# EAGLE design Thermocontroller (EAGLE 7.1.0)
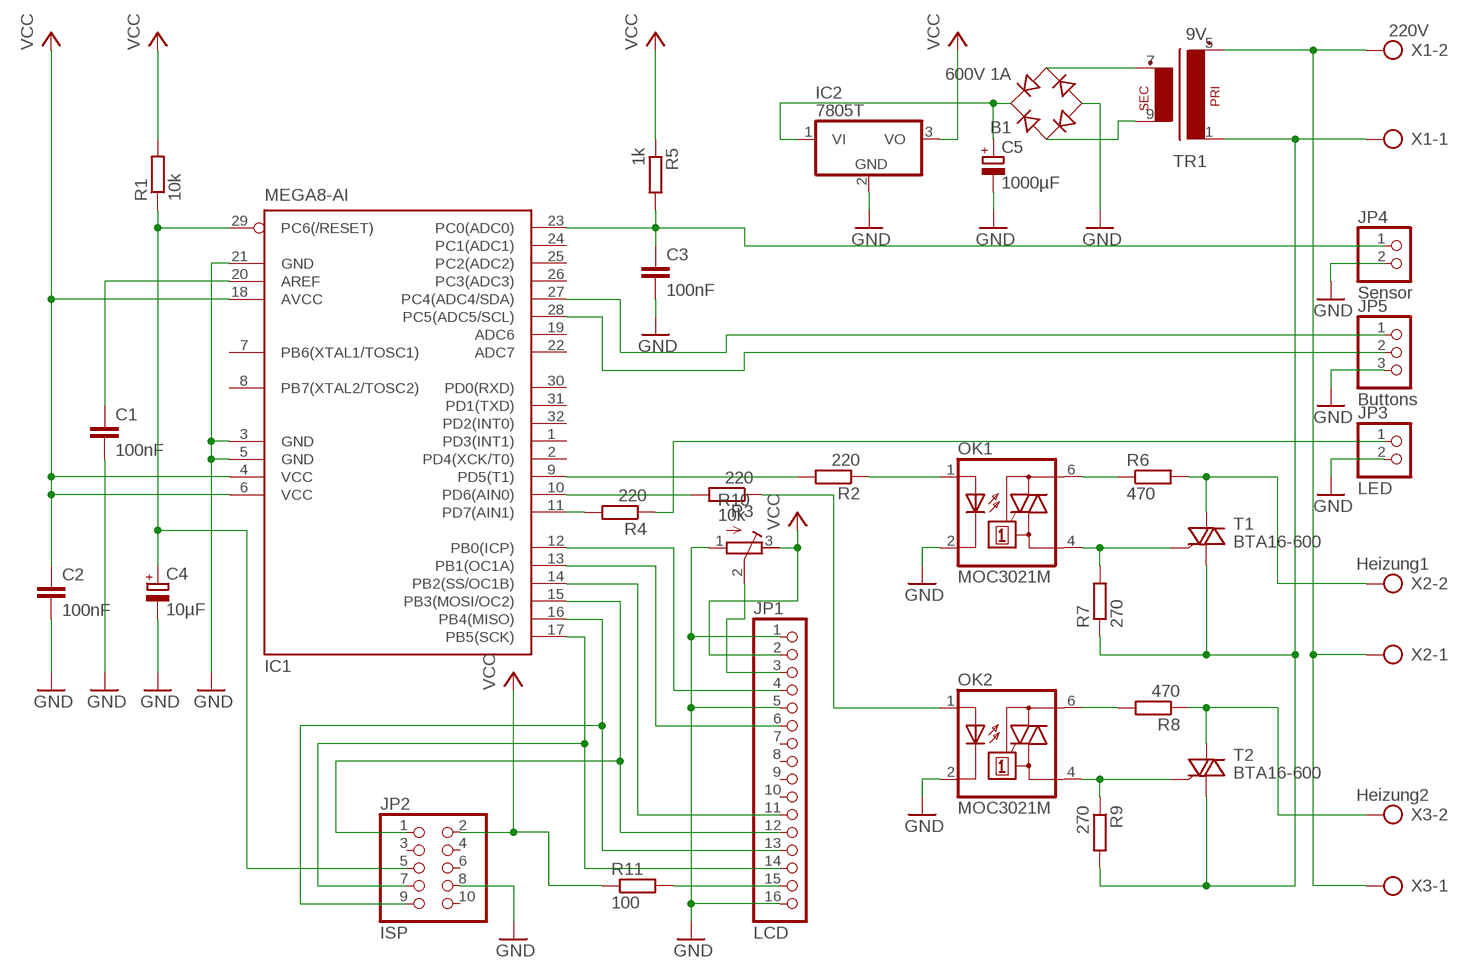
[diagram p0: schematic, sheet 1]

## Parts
B1  600V 1A  RB1A  [RB1A]
C1  100nF  C-EUC1206  [C1206]
C2  100nF  C-EUC0805  [C0805]
C3  100nF  C-EUC0805  [C0805]
C4  10µF  CPOL-EUSMCB  [SMC_B]
C5  1000µF  CPOL-EUE7.5-16  [E7,5-16]
IC1  MEGA8-AI  [TQFP32-08]
IC2  7805T  [TO220H]
JP1  LCD  PINHD-1X16  [1X16]
JP2  ISP  PINHD-2X5  [2X05]
JP3  LED  PINHD-1X2  [1X02]
JP4  Sensor  PINHD-1X2  [1X02]
JP5  Buttons  PINHD-1X3  [1X03]
OK1  MOC3021M  [DIL06]
OK2  MOC3021M  [DIL06]
R1  10k  R-EU_R1206  [R1206]
R2  220  R-EU_R1206  [R1206]
R3  220  R-EU_R1206  [R1206]
R4  220  R-EU_R1206  [R1206]
R5  1k  R-EU_R1206  [R1206]
R6  470  R-EU_0207/10  [0207/10]
R7  270  R-EU_0207/10  [0207/10]
R8  470  R-EU_0207/10  [0207/10]
R9  270  R-EU_0207/10  [0207/10]
R10  10k  R-TRIMM64Y  [RTRIM64Y]
R11  100  R-EU_0207/10  [0207/10]
T1  BTA16-600  BT138-V  [TO220BV]
T2  BTA16-600  BT138-V  [TO220BV]
TR1  9V  EI30-1  [EI30-1]
X1  220V  AK500/2  [AK500/2]
X2  Heizung1  AK500/2  [AK500/2]
X3  Heizung2  AK500/2  [AK500/2]

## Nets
GND: B1.- C1.2 C2.2 C3.2 C4.- C5.- IC1.3(GND) IC1.5(GND) IC1.21(GND) IC2.2(GND) JP1.1 JP1.5 JP1.16 JP2.8 JP3.2 JP4.2 JP5.3 OK1.2(C) OK2.2(C) R10.1(A)
N$1: TR1.5(P2) X1.2 X2.1 X3.1
N$2: B1.AC2 TR1.7(S3)
N$4: B1.AC1 TR1.9(S4)
N$5: B1.+ C5.+ IC2.1(VI)
N$6: OK2.6(A2) R8.2
N$7: OK1.6(A2) R6.1
N$8: OK2.4(A1) R9.1 T2.G
N$9: OK1.4(A1) R7.2 T1.G
N$13: R8.1 T2.T2(A2) X3.2
N$14: OK1.1(A) R2.1
N$15: IC1.9(PD5(T1)) R2.2
N$16: IC1.10(PD6(AIN0)) R3.2
N$17: OK2.1(A) R3.1
N$18: JP3.1 R4.1
N$19: IC1.11(PD7(AIN1)) R4.2
N$20: IC1.17(PB5(SCK)) JP1.14 JP2.7
N$21: IC1.16(PB4(MISO)) JP1.13 JP2.9
N$22: IC1.15(PB3(MOSI/OC2)) JP1.12 JP2.1
N$23: IC1.14(PB2(SS/OC1B)) JP1.11
N$24: IC1.13(PB1(OC1A)) JP1.6
N$25: IC1.12(PB0(ICP)) JP1.4
N$26: C3.1 IC1.23(PC0(ADC0)) JP4.1 R5.2
N$27: IC1.27(PC4(ADC4/SDA)) JP5.1
N$28: IC1.28(PC5(ADC5/SCL)) JP5.2
N$29: R7.1 R9.2 T1.T1(A1) T2.T1(A1) TR1.1 X1.1
N$30: C1.1 IC1.20(AREF)
N$31: C4.+ IC1.29(PC6(/RESET)) JP2.5 R1.1
N$32: R6.2 T1.T2(A2) X2.2
N$35: JP1.3 R10.2(S)
N$38: JP1.15 R11.2
VCC: C2.1 IC1.4(VCC) IC1.6(VCC) IC1.18(AVCC) IC2.3(VO) JP1.2 JP2.2 R1.2 R5.1 R10.3(E) R11.1
Unconnected: IC1.1(PD3(INT1)) IC1.2(PD4(XCK/T0)) IC1.7(PB6(XTAL1/TOSC1)) IC1.8(PB7(XTAL2/TOSC2)) IC1.19(ADC6) IC1.22(ADC7) IC1.24(PC1(ADC1)) IC1.25(PC2(ADC2)) IC1.26(PC3(ADC3)) IC1.30(PD0(RXD)) IC1.31(PD1(TXD)) IC1.32(PD2(INT0)) JP1.7 JP1.8 JP1.9 JP1.10 JP2.3 JP2.4 JP2.6 JP2.10

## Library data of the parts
B1 = rectifier:RB1A: RECTIFIER 1 A
C1-C3 = rcl:C-EU: CAPACITOR, European symbol
C4 C5 = rcl:CPOL-EU: POLARIZED CAPACITOR, European symbol
IC1 = atmel:MEGA8: MICROCONTROLLER 8 Kbytes FLASH, 1 kbytes SRAM, 512 bytes EEPROM, USART, 6-channel 10 bit ADC, 2-channel 8 bit ADC Pin compatible with Atmega48, ATMega88, ATMega168 Source: avr.lbr; MPN: ATMEGA8-16AU; OC_FARNELL: 9171371; OC_NEWARK: 73M8863
IC2 = linear:78*: Positive VOLTAGE REGULATOR Source: http://cache.national.com/ds/LM/LM78L05.pdf http://www.fairchildsemi.com/ds/LM/LM7805.pdf
JP1 = pinhead:PINHD-1X16: PIN HEADER
JP2 = pinhead:PINHD-2X5: PIN HEADER
JP3 JP4 = pinhead:PINHD-1X2: PIN HEADER
JP5 = pinhead:PINHD-1X3: PIN HEADER
OK1 OK2 = optocoupler:MOC30*M: RANDOM-PHASE OPTOISOLATORS TRIAC DRIVER OUTPUT Source: http://www.fairchildsemi.com MOC3020-M.pdf; MF: FAIRCHILD SEMICONDUCTOR; MPN: MOC3021-M; OC_FARNELL: 1021365; OC_NEWARK: 95B7895
R1-R9 R11 = rcl:R-EU_: RESISTOR, European symbol
R10 = rcl:R-TRIMM: Trimm resistor
T1 T2 = triac:BT138: TRIAC Source: http://www.semiconductors.philips.com BT138_SERIES_2.pdf
TR1 = trafo:EI30-1: TRANSFORMER 1 primary winding, 1 secondary winding ERA
X1-X3 = con-ptr500:AK500/2: CONNECTOR; OC_FARNELL: unknown; OC_NEWARK: unknown

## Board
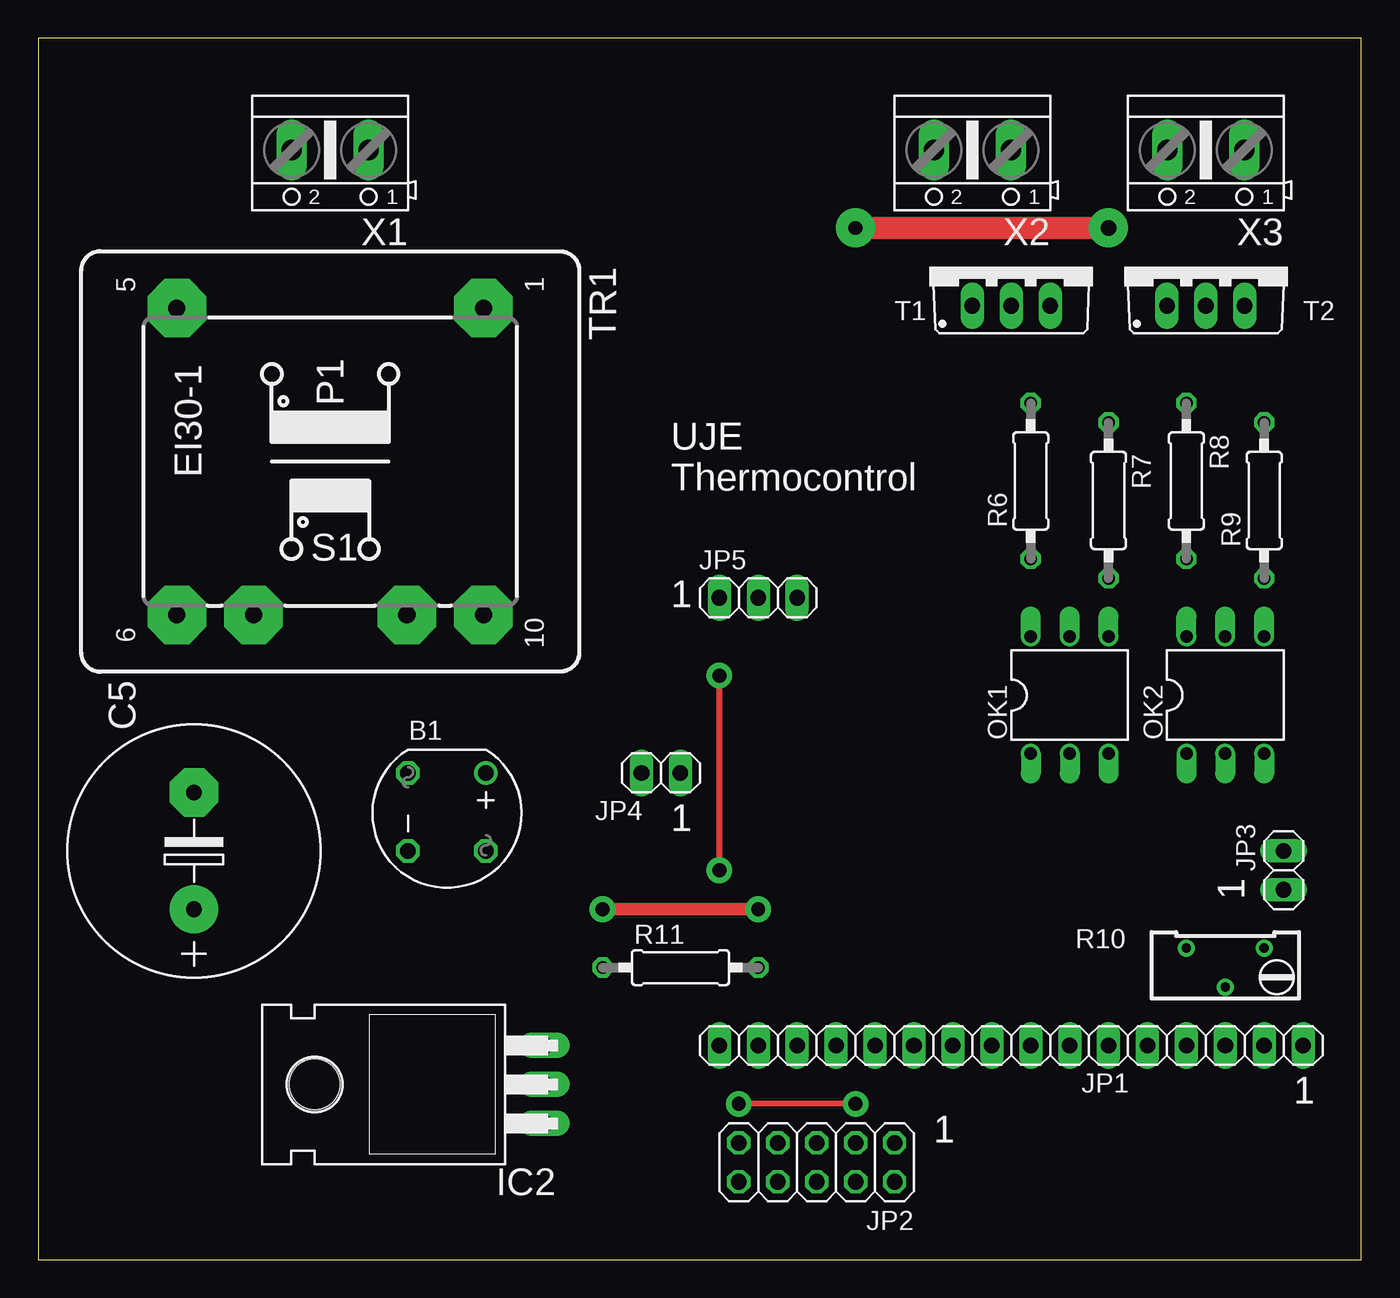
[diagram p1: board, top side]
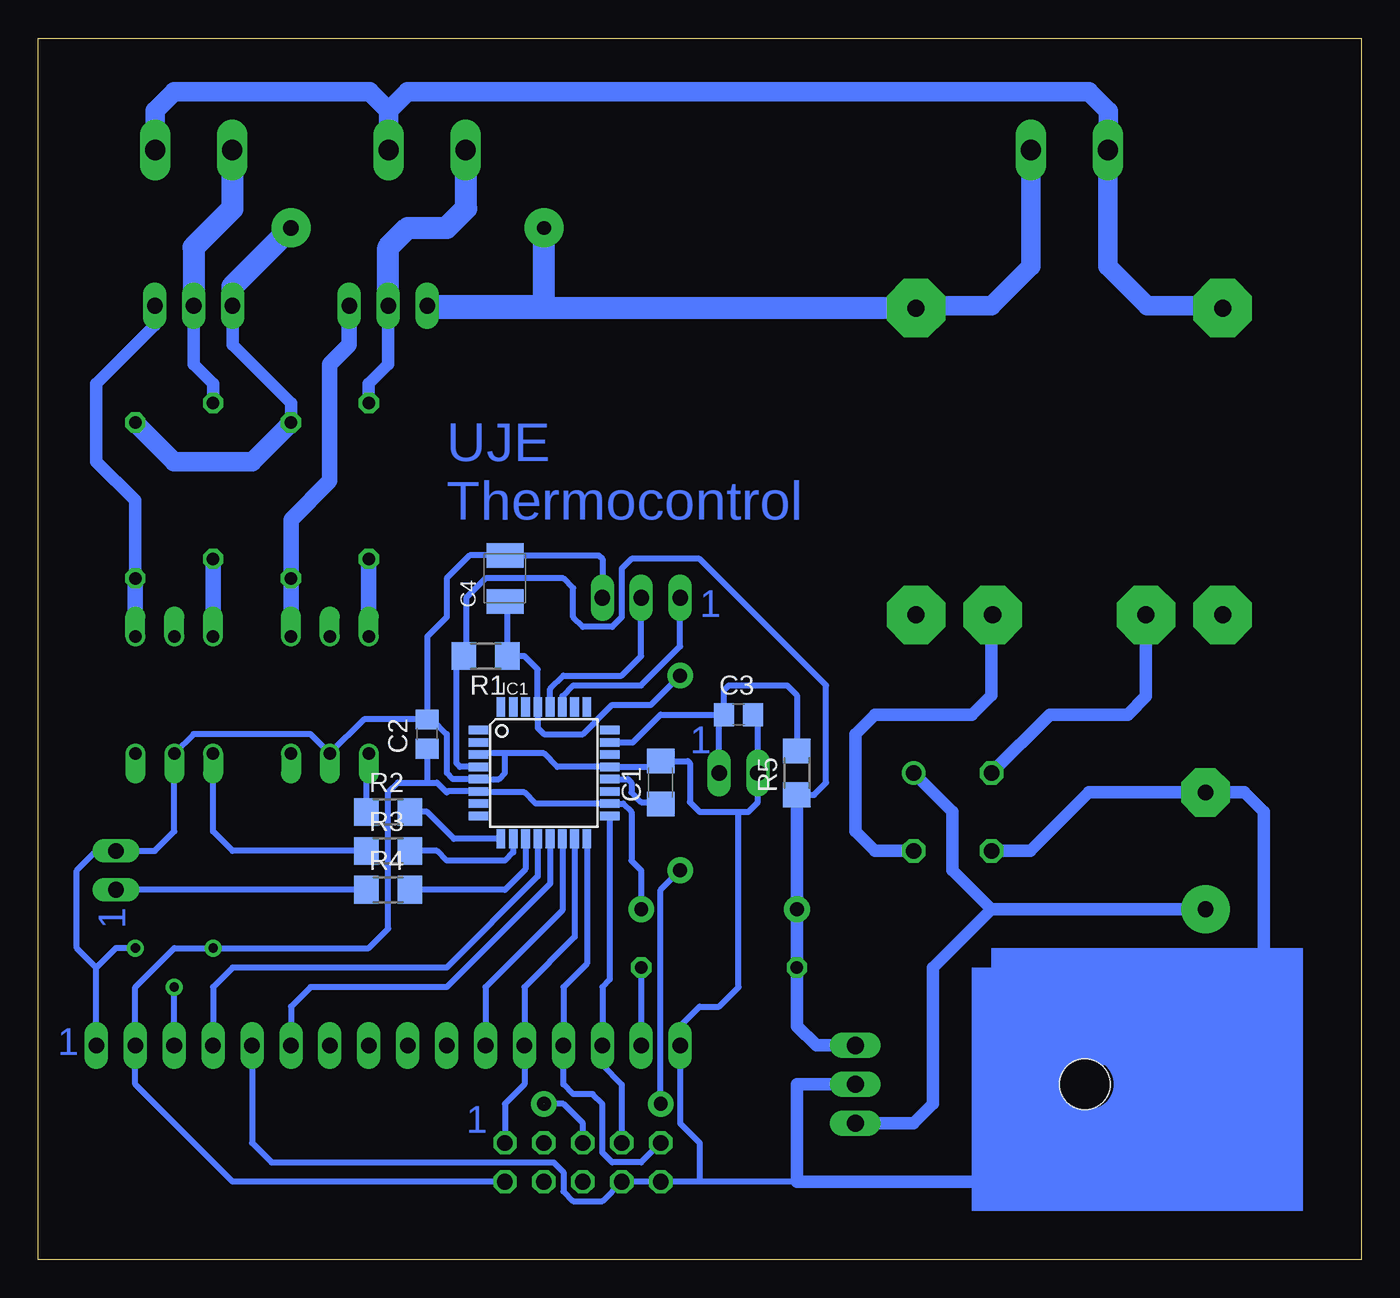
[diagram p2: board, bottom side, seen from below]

Size 86.34 x 79.68 mm. Coordinates in mm from the lower left corner, seen from the top.
Outline: 0,0 86.34,0 86.34,79.68 0,79.68 0,0
Copper layers (1*16): Top 0.035mm / dielectric 1.5mm / Bottom 0.035mm
Design rules "default": minimum track width 10mil, minimum drill 24mil, track to track 8mil, track to pad 8mil, pad to pad 8mil, via to via 8mil, smd to smd 8mil, copper to edge 40mil, drill to drill 8mil, minimum pad ring 10mil, minimum via ring 8mil, stop-mask expansion 4mil, vias tented up to drill 0mil, thermal gap 10mil

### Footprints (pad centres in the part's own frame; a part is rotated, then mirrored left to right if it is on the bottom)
RB1A = drill 1.016: + -2.54,2.54 | drill 1.016 octagon: - 2.54,-2.54; AC1 2.54,2.54; AC2 -2.54,-2.54
C1206 = smd 1.6 x 1.8: 1 -1.4,0; 2 1.4,0
C0805 = smd 1.3 x 1.5: 1 -0.95,0; 2 0.95,0
SMC_B = smd 1.6 x 2.4: + -1.5,0; - 1.5,0
E7,5-16 = drill 1.016 pad 3.15: + -3.81,0 | drill 1.016 pad 3.15 octagon: - 3.81,0
TQFP32-08 = smd 1.27 x 0.559: 1 -4.293,2.8; 2 -4.293,2; 3 -4.293,1.2; 4 -4.293,0.4; 5 -4.293,-0.4; 6 -4.293,-1.2; 7 -4.293,-2; 8 -4.293,-2.8; 17 4.293,-2.8; 18 4.293,-2; 19 4.293,-1.2; 20 4.293,-0.4; 21 4.293,0.4; 22 4.293,1.2; 23 4.293,2; 24 4.293,2.8 | smd 0.559 x 1.27: 9 -2.8,-4.293; 10 -2,-4.293; 11 -1.2,-4.293; 12 -0.4,-4.293; 13 0.4,-4.293; 14 1.2,-4.293; 15 2,-4.293; 16 2.8,-4.293; 25 2.8,4.293; 26 2,4.293; 27 1.2,4.293; 28 0.4,4.293; 29 -0.4,4.293; 30 -1.2,4.293; 31 -2,4.293; 32 -2.8,4.293
TO220H = drill 1.118 long: 1 -2.54,-10.16; 2 0,-10.16; 3 2.54,-10.16 | hole 3.302: 0,4.826
1X16 = drill 1.016 long: 1 -19.05,0; 2 -16.51,0; 3 -13.97,0; 4 -11.43,0; 5 -8.89,0; 6 -6.35,0; 7 -3.81,0; 8 -1.27,0; 9 1.27,0; 10 3.81,0; 11 6.35,0; 12 8.89,0; 13 11.43,0; 14 13.97,0; 15 16.51,0; 16 19.05,0
2X05 = drill 1.016 octagon: 1 -5.08,-1.27; 2 -5.08,1.27; 3 -2.54,-1.27; 4 -2.54,1.27; 5 0,-1.27; 6 0,1.27; 7 2.54,-1.27; 8 2.54,1.27; 9 5.08,-1.27; 10 5.08,1.27
1X02 = drill 1.016 long: 1 -1.27,0; 2 1.27,0
1X03 = drill 1.016 long: 1 -2.54,0; 2 0,0; 3 2.54,0
DIL06 = drill 0.813 offset: 1 -2.54,-3.81; 2 0,-3.81; 3 2.54,-3.81; 4 2.54,3.81; 5 0,3.81; 6 -2.54,3.81
R1206 = smd 1.6 x 1.803: 1 -1.422,0; 2 1.422,0
0207/10 = drill 0.813 octagon: 1 -5.08,0; 2 5.08,0
RTRIM64Y = drill 0.61: 1 0,-2.54; 2 -2.54,0; 3 0,2.54
TO220BV = drill 1.016 long: G 2.54,-2.54; T1 -2.54,-2.54; T2 0,-2.54
EI30-1 = drill 1.118 pad 3.81 octagon: 1 -10.008,10.008; 5 -10.008,-10.008; 6 10.008,-10.008; 7 10.008,-5.004; 9 10.008,5.004; 10 10.008,10.008
AK500/2 = drill 1.321 long: 1 -2.515,0; 2 2.515,0

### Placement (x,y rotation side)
B1  26.67,29.21 270 top
C1  45.72,31.12 90 bottom
C2  60.96,34.29 90 bottom
C3  40.64,35.56 0 bottom
C4  55.88,44.45 90 bottom
C5  10.16,26.67 90 top
IC1  53.34,31.75 0 bottom
IC2  22.86,11.43 90 top
JP1  63.5,13.97 180 top
JP2  50.8,6.35 180 top
JP3  81.28,25.4 90 top
JP4  40.64,31.75 180 top
JP5  46.99,43.18 0 top
OK1  67.31,36.83 0 top
OK2  77.47,36.83 0 top
R1  57.15,39.37 180 bottom
R2  63.5,29.21 0 bottom
R3  63.5,26.67 0 bottom
R4  63.5,24.13 0 bottom
R5  36.83,31.75 90 bottom
R6  64.77,50.8 90 top
R7  69.85,49.53 270 top
R8  74.93,50.8 270 top
R9  80.01,49.53 90 top
R10  77.47,20.32 90 top
R11  41.91,19.05 0 top
T1  63.5,64.77 0 top
T2  76.2,64.77 0 top
TR1  19.05,52.07 270 top
X1  19.05,72.39 180 top
X2  60.96,72.39 180 top
X3  76.2,72.39 180 top

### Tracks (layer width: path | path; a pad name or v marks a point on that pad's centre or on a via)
GND
  Bottom 0.406: JP1.1 82.55,19.05 | 82.55,19.05 83.82,20.32 83.82,25.4 82.55,26.67 JP3.2 78.74,26.67 77.47,27.94 OK2.2 76.2,34.29 68.58,34.29 OK1.2 65.09,35.24 C2.2 | R10.1 81.28,20.32 82.55,19.05 | 55.88,33.02 53.34,33.02 52.47,32.15 IC1.21 46.09,32.15 C1.2 43.95,32.52 43.81,32.38 43.81,29.84 43.18,29.21 40.64,29.21 | 55.88,33.02 57.56,33.02 IC1.3 | C2.2 60.64,35.24 59.69,34.29 59.69,31.75 59.29,31.35 IC1.5 56.28,31.35 55.88,31.75 55.88,33.02 | C2.2 60.96,40.64 59.69,41.91 59.69,44.45 58.19,45.95 C4.- 49.76,45.95 49.53,45.72 JP5.3 | 36.83,5.08 43.18,5.08 | 43.18,5.08 JP2.8 49.53,3.81 51.44,3.81 52.07,4.45 52.07,5.71 52.7,6.35 71.12,6.35 72.39,7.62 JP1.5 | C3.2 39.37,35.24 JP4.2 39.37,29.84 40.01,29.21 40.64,29.21 | 43.18,5.08 43.18,7.62 44.45,8.89 JP1.16 44.45,15.24 43.18,16.51 41.91,16.51 40.64,17.78 40.64,29.21
  Bottom 0.813: B1.- 21.59,26.67 17.78,30.48 C5.- 7.62,30.48 6.35,29.21 6.35,7.62 8.89,5.08 36.83,5.08 36.83,11.43 IC2.2
N$1
  Bottom 1.27: TR1.5 9.2,62.23 13.97,62.23 16.54,64.8 X1.2 16.51,72.42 16.51,74.93 17.78,76.2 62.23,76.2 63.48,74.95 | X2.1 63.48,74.95 | X3.1 78.72,74.95 77.47,76.2 64.72,76.2 63.48,74.95
N$2
  Bottom 0.813: TR1.7 14.05,36.75 15.24,35.56 20.32,35.56 B1.AC2
N$3  (via drill 0.9 pad 1.68)
  other vias: 53.34,10.16
N$4
  Bottom 0.813: B1.AC1 31.75,26.67 33.02,27.94 33.02,34.29 31.75,35.56 25.4,35.56 24.13,36.83 24.13,41.99 TR1.9
N$5
  Bottom 0.813: B1.+ 26.67,29.21 26.67,25.4 24.13,22.86 | 24.13,22.86 C5.+ | 24.13,22.86 27.94,19.05 27.94,10.16 29.21,8.89 IC2.1
N$6
  Bottom 1.016: OK2.6 R8.2
N$7
  Bottom 1.016: OK1.6 R6.1
N$8
  Bottom 0.813: R9.1 80.01,49.53 82.55,52.07 82.55,57.15 78.74,60.96 T2.G
  Bottom 1.016: OK2.4 R9.1
N$9
  Bottom 1.016: OK1.4 R7.2 69.85,48.26 67.31,50.8 67.31,58.42 66.04,59.69 T1.G
N$10  (via drill 1 pad 2.54)
  other vias: 69.85,67.31
N$11  (via drill 0.9 pad 2.54)
  other vias: 53.34,67.31
N$13
  Bottom 0.813: T2.T2 76.2,58.42 74.93,57.15 R8.1
  Bottom 1.27: 73.66,72.36 X3.2
  Bottom 1.422: X3.2 73.69,68.56 76.2,66.04 T2.T2
N$14
  Bottom 0.406: R2.1 64.92,32.87 OK1.1
N$15
  Bottom 0.406: IC1.9 59.21,27.46 60.96,29.21 R2.2
N$16
  Bottom 0.406: IC1.10 55.34,26.58 55.88,26.04 59.69,26.04 60.33,26.67 R3.2
N$17
  Bottom 0.406: R3.1 73.66,26.67 74.93,27.94 OK2.1
N$18
  Bottom 0.406: R4.1 JP3.1
N$19
  Bottom 0.406: IC1.11 54.54,25.47 55.88,24.13 R4.2
N$20
  Bottom 0.406: IC1.17 49.05,18.26 49.53,17.78 JP1.14 49.53,12.7 48.26,11.43 JP2.7
N$21
  Bottom 0.406: IC1.16 50.54,19.31 52.07,17.78 JP1.13 52.07,11.43 51.44,10.8 50.16,10.8 49.53,10.16 49.53,6.98 48.9,6.35 46.99,6.35 JP2.9
N$22
  Bottom 0.406: IC1.15 51.34,21.05 54.61,17.78 JP1.12 54.61,11.43 55.88,10.16 JP2.1
N$23
  Bottom 0.406: IC1.14 52.14,22.79 57.15,17.78 JP1.11
N$24
  Bottom 0.406: IC1.13 52.94,24.53 59.69,17.78 68.58,17.78 69.85,16.51 JP1.6
N$25
  Bottom 0.406: IC1.12 53.74,25 59.69,19.05 73.66,19.05 74.93,17.78 JP1.4
N$26
  Bottom 0.406: IC1.23 47.53,33.75 45.72,35.56 C3.1 | JP4.1 41.91,35.24 C3.1 | C3.1 41.59,37.15 41.27,37.47 37.47,37.47 36.83,36.83 R5.2
N$27
  Bottom 0.406: IC1.27 52.14,36.76 51.44,37.47 46.99,37.47 44.45,40.01 JP5.1
N$28
  Bottom 0.406: IC1.28 52.94,37.23 52.07,38.1 48.26,38.1 46.99,39.37 JP5.2
N$29
  Top 1.422: 53.34,67.31 69.85,67.31
  Bottom 0.813: R7.1 69.85,55.88 73.66,59.69 T2.T1
  Bottom 1.27: X1.1 21.57,64.8 24.13,62.23 28.91,62.23 TR1.1 | R9.2 77.47,52.07 72.39,52.07 R7.1
  Bottom 1.422: T2.T1 73.66,63.5 69.85,67.31 | 53.34,67.31 53.34,62.23 T1.T1 60.81,62.08 TR1.1
N$30
  Bottom 0.406: IC1.20 47.86,31.35 47.62,31.12 47.62,30.48 46.99,29.84 45.85,29.84 C1.1
N$31  (via drill 0.9 pad 1.68)  (1 unrouted)
  Top 0.406: 53.34,10.16 v45.72,10.16 | v44.45,25.4 v44.45,38.1
  Bottom 0.406: C4.+ 55.73,42.8 R1.1 54.61,39.37 53.74,38.5 IC1.29 53.74,34.69 53.34,34.29 50.8,34.29 48.9,36.2 46.35,36.2 v44.45,38.1 | JP2.5 50.8,8.89 52.07,10.16 53.34,10.16 | v45.72,10.16 45.72,24.13 v44.45,25.4
N$32
  Bottom 0.813: T1.T2 63.5,58.42 64.77,57.15 R6.2
  Bottom 1.422: T1.T2 63.5,66.04 62.23,67.31 59.69,67.31 58.42,68.58 58.42,72.36 X2.2
N$35
  Bottom 0.406: JP1.3 R10.2
N$38
  Bottom 0.406: R11.2 JP1.15
VCC  (via drill 0.9 pad 1.68)
  Top 0.813: v36.83,22.86 v46.99,22.86
  Bottom 0.406: 60.96,31.12 62.87,31.12 63.5,30.48 63.5,21.59 64.77,20.32 R10.3 77.47,20.32 80.01,17.78 JP1.2 80.01,11.43 73.66,5.08 JP2.2 | 60.96,31.12 60.33,31.12 59.69,30.48 59.62,30.55 IC1.6 57.56,30.48 54.61,30.48 53.88,29.75 IC1.18 48.16,29.75 47.62,29.21 47.62,26.04 46.99,25.4 v46.99,22.86 | IC1.4 58.82,32.15 59.05,32.38 59.05,38.89 R1.2 58.42,39.52 58.42,43.18 57.15,44.45 52.07,44.45 51.44,43.81 51.44,41.91 50.8,41.28 48.9,41.28 48.26,41.91 48.26,45.08 47.62,45.72 43.18,45.72 34.92,37.47 34.92,31.12 35.71,30.33 R5.1 | C2.1 60.96,31.12
  Bottom 0.813: IC2.3 35.56,13.97 36.83,15.24 R11.1 v36.83,22.86 R5.1
(copper drawn outside any net)
  shapes: Bottom area x7, Bottom circle x1

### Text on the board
Bottom: UJE / Thermocontrol | 1 | 1 | 1 | 1 | 1
tNames: UJE / Thermocontrol | 1 | 1 | 1 | 1 | 1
